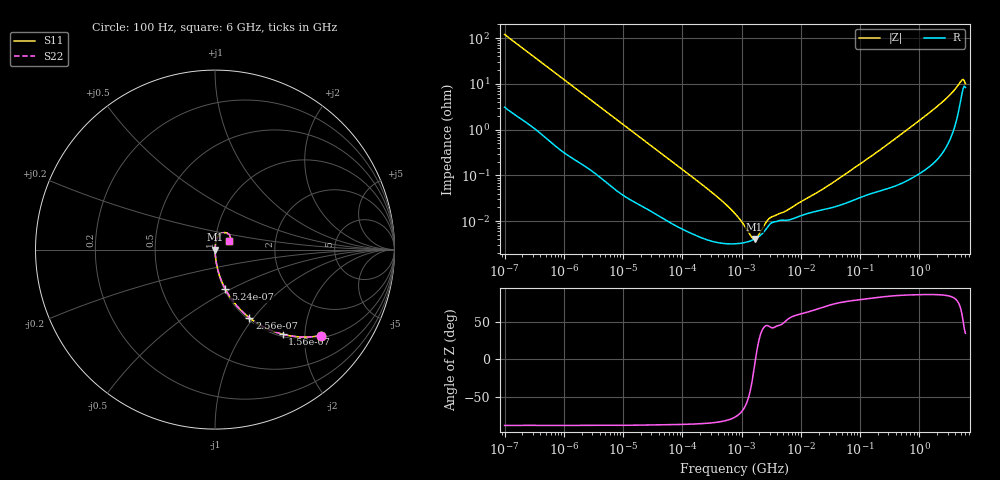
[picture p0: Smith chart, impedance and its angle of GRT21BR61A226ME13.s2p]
!Murata Part Number: GRT21BR61A226ME13
!These Parameters are Measured in Series Mode Connection
!Data Generated on Jun 19, 2026
!  o--ll--o
!Port1  Port2
!  o------o
!Operation Temp=25[degC], DC Bias Voltage=0[V]
!Freq. Start=100[Hz] Stop=6[GHz] 401[Steps]
# Hz S RI R 50
!Freq.(Hz) S11(Real) S11(Imag) S21(Real) S21(Imag) S12(Real) S12(Imag) S22(Real) S22(Imag)
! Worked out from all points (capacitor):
!   401 points, 100 Hz to 6 GHz, reference 50 ohm
!   read as one part in series: C = 13.2 uF near 109 Hz
!   lowest |Z| = 4.1 mohm at 1.658 MHz (marker M1)
!   series resonance near 1.72 MHz, so ESL is about 650 pH
!   S11 on the Smith chart (normalised r, x): 100 Hz: 1.06, -2.40; 156 Hz: 1.04, -1.54; 256 Hz: 1.03, -0.95; 524 Hz: 1.01, -0.47; 6 GHz: 1.17, +0.11
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100  0.5885 -0.4794  0.4115 0.4794  0.4115 0.4794  0.5885 -0.4794
156  0.377 -0.4717  0.623 0.4717  0.623 0.4717  0.377 -0.4717
256  0.1915 -0.38  0.8085 0.38  0.8085 0.38  0.1915 -0.38
524  0.0579 -0.2208  0.9421 0.2208  0.9421 0.2208  0.0579 -0.2208
981  0.019 -0.1243  0.981 0.1243  0.981 0.1243  0.019 -0.1243
2008  0.00566 -0.0623  0.9943 0.0623  0.9943 0.0623  0.00566 -0.0623
40335  0.000141 -0.0033  0.9999 0.0033  0.9999 0.0033  0.000141 -0.0033
316350  3.66e-05 -0.000424  1 0.000424  1 0.000424  3.66e-05 -0.000424
774597  3.22e-05 -0.000144  1 0.000144  1 0.000144  3.22e-05 -0.000144
926525  3.28e-05 -0.000107  1 0.000107  1 0.000107  3.28e-05 -0.000107
1059725  3.36e-05 -8.19e-05  1 8.19e-05  1 8.19e-05  3.36e-05 -8.19e-05
1658239  4.06e-05 -5.9e-06  1 5.9e-06  1 5.9e-06  4.06e-05 -5.9e-06
2594782  6.73e-05 6.67e-05  0.9999 -6.67e-05  0.9999 -6.67e-05  6.73e-05 6.67e-05
3245845  9.32e-05 8.34e-05  0.9999 -8.34e-05  0.9999 -8.34e-05  9.32e-05 8.34e-05
5809218  0.000105 0.000136  0.9999 -0.000136  0.9999 -0.000136  0.000105 0.000136
1.555665e7  0.000158 0.000332  0.9998 -0.000332  0.9998 -0.000332  0.000158 0.000332
3.983537e7  0.000212 0.000757  0.9998 -0.000757  0.9998 -0.000757  0.000212 0.000757
3.124326e8  0.000555 0.00507  0.9994 -0.00507  0.9994 -0.00507  0.000555 0.00507
2.240541e9  0.00392 0.0361  0.9961 -0.0361  0.9961 -0.0361  0.00392 0.0361
3.352442e9  0.0097 0.0577  0.9903 -0.0577  0.9903 -0.0577  0.0097 0.0577
5.016141e9  0.0523 0.0951  0.9477 -0.0951  0.9477 -0.0951  0.0523 0.0951
6e9  0.0797 0.0488  0.9203 -0.0488  0.9203 -0.0488  0.0797 0.0488
